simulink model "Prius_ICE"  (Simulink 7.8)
settings: Solver=ode23tb  StartTime=0.0  StopTime=1180  RelTol=1e-3
InitFcn:
  | init_Prius_GT
StopFcn:
  | Vyhodnoceni
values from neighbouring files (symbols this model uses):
  om_diff_ic = 0    [init_Prius_GT.m]
  omric = 0    [init_Prius_GT.m]
  rpm_FMEP = [1,500,1000,1500,2000,2500,3000,3500,4000,4500,5000]    [init_Prius_GT.m]
  t_sample = 0.1    [init_Prius_GT.m]
  torque_FMEP = [0,0,0.58,0.66,0.75,0.84,0.93,1.1,1.3,1.4,1.5].*(Vdis/(4*pi))*100000    [init_Prius_GT.m]
  vf0 = 0    [init_Prius_GT.m]
undefined symbols (not defined in the file or in its folder): Clutch, Control, Differential, Driveshaft, Engine, Environment, Gearbox, Powertrain, table_FMEP, Vehicle
libraries: simulink x30, simulink_extras x6, simulink_need_slupdate x1
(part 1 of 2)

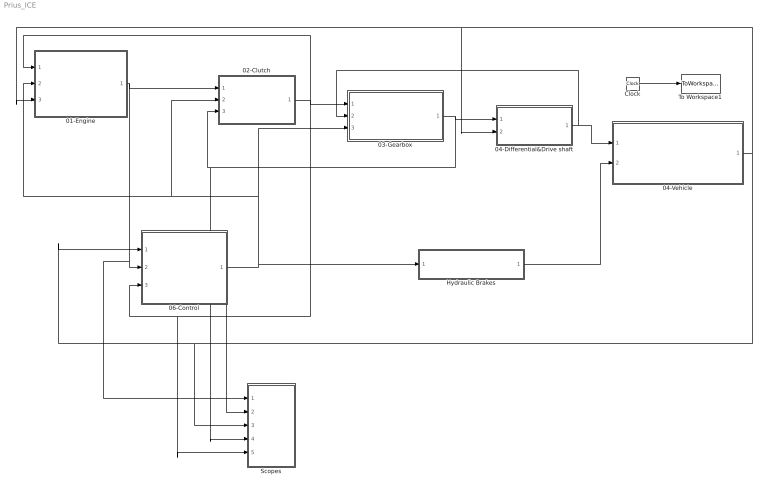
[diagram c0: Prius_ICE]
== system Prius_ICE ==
  01-Engine : Subsystem  AncestorBlock=Powertrain/01-Engine
  02-Clutch : Subsystem  AncestorBlock=Powertrain/02-Clutch
  03-Gearbox : Subsystem  AncestorBlock=Powertrain/03-Gearbox
  04-Differential&Drive shaft : Subsystem  AncestorBlock=Powertrain/04-Differential&Drive shaft
  04-Vehicle : Subsystem  AncestorBlock=Powertrain/05-Vehicle
  06-Control : Subsystem  AncestorBlock=Powertrain/06-Control
  Clock : Clock
  Hydraulic Brakes : Subsystem  AncestorBlock=Powertrain/Hydraulic Brakes  TreatAsAtomicUnit=on
  Scopes : Subsystem  AncestorBlock=Powertrain/Scopes
  To Workspace1 : ToWorkspace  VariableName=t  SampleTime=t_sample  SaveFormat=Array
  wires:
  01-Engine/1(BUS_Engine) -> 02-Clutch/1(BUS_Engine), 06-Control/2(BUS_Engine), Scopes/1(BUS_Engine)
  02-Clutch/1(BUS_Clutch) -> 03-Gearbox/1(BUS_Clutch), 01-Engine/1(BUS_Clutch), 06-Control/3(BUS_Clutch), Scopes/5(BUS_Clutch)
  03-Gearbox/1(BUS_Gearbox) -> 04-Differential&Drive shaft/1(BUS_Gearbox), 02-Clutch/3(BUS_Gearbox), Scopes/4(BUS_Gearbox)
  04-Differential&Drive shaft/1(BUS_Driveshaft) -> 03-Gearbox/2(BUS_Driveshaft), 04-Vehicle/1(BUS_Driveshaft_Front)
  06-Control/1(BUS_Control) -> Scopes/2(BUS_Control), 01-Engine/2(BUS_Control), 02-Clutch/2(BUS_Control), 03-Gearbox/3(BUS_Control), Hydraulic Brakes/1(BUS_Control)
  04-Vehicle/1(BUS_Vehicle) -> 06-Control/1(BUS_Vehicle), Scopes/3(BUS_Vehicle), 01-Engine/3(BUS_vehicle), 04-Differential&Drive shaft/2(BUS_Vehicle)
  Hydraulic Brakes/1(BUS_Brakes) -> 04-Vehicle/2(BUS_Brakes)
  Clock/1 -> To Workspace1/1

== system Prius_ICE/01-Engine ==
  note: Tec[Nm]
  BUS_Clutch : Inport
  BUS_Control : Inport  Port=2
  BUS_vehicle : Inport  Port=3
  1-D Lookup Table : Lookup_n-D  NumberOfTableDimensions=1  BreakpointsForDimension1=[1000,1625,2250,3000,3750,4500,5250,5625]  Table=[85,90,100,112,100,92,85,78]  RndMeth=Simplest
  Bus Creator : BusCreator  Inputs=5
  Bus Selector : BusSelector  OutputSignals=om_fric1
  Bus Selector1 : BusSelector  OutputSignals=Throttle_pedal[-],Status_Num
  Bus Selector2 : BusSelector  OutputSignals=s_veh
  Consumption/Emissions : Subsystem
  Display : Display
  Idling PID : Subsystem
  Mechanical1 : Subsystem
  Product2 : Product
  Saturation : Saturate  UpperLimit=inf  LowerLimit=0
  Scope : Scope  NumInputPorts=3
  rad2rpm : Gain  Gain=30/pi
  BUS_Engine : Outport
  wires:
  Idling PID/1(Te_dem) -> Mechanical1/1(Te_dem)
  1-D Lookup Table/1 -> Product2/1
  Product2/1 -> Idling PID/1(Te), Scope/3
  Bus Selector1/1 -> Scope/1, Product2/2  "<Throttle_pedal[-]>"
  Consumption/Emissions/2(Fuel_cons_m) -> Bus Creator/5  "Fuel_cons_m"
  Saturation/1 -> Consumption/Emissions/2(Pe)
  Consumption/Emissions/1(Fuel_cons) -> Bus Creator/4  "fuel_cons [l_100km]"
  Bus Selector2/1 -> Display/1, Consumption/Emissions/3(s)  "<s_veh>"
  BUS_vehicle/1 -> Bus Selector2/1
  BUS_Control/1 -> Bus Selector1/1
  Bus Selector/1 -> Mechanical1/2(om_fric)  "<om_fric1>"
  BUS_Clutch/1 -> Bus Selector/1
  Bus Creator/1 -> BUS_Engine/1
  Mechanical1/3(Tec) -> Bus Creator/3, Consumption/Emissions/4(Te)
  Mechanical1/2(Pe) -> Saturation/1, Bus Creator/2  "Pe[kW]"
  Mechanical1/1(om_e) -> rad2rpm/1
  rad2rpm/1 -> Scope/2, 1-D Lookup Table/1, Idling PID/2(n_eng[rpm]), Bus Creator/1, Consumption/Emissions/1(n_eng[rpm])  "n_eng[rpm]"

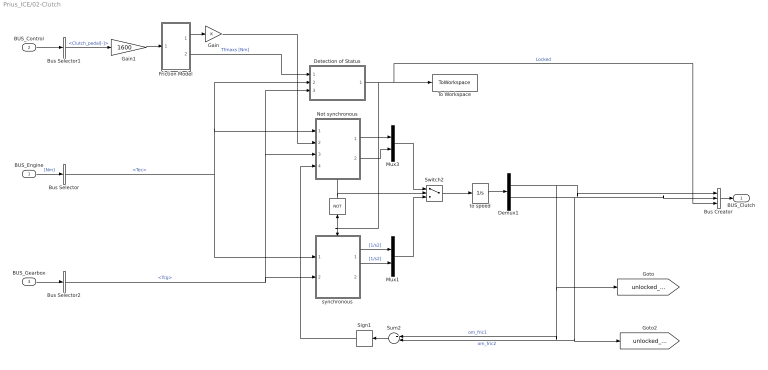
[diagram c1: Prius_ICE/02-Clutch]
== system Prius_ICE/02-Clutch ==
  BUS_Engine : Inport
  BUS_Control : Inport  Port=2
  BUS_Gearbox : Inport  Port=3
  " " : Logic  Operator=NOT  Inputs=1
  Bus Creator : BusCreator  Inputs=3
  Bus Selector : BusSelector  OutputSignals=Tec
  Bus Selector1 : BusSelector  OutputSignals=Clutch_pedal[-]
  Bus Selector2 : BusSelector  OutputSignals=Tcg
  Demux1 : Demux  Outputs=2
  Detection of Status : Subsystem
  Friction Model : Subsystem
  Gain : Gain
  Gain1 : Gain  Gain=1600
  Mux1 : Mux  Inputs=2
  Mux3 : Mux  Inputs=2
  Not synchronous : Subsystem  TreatAsAtomicUnit=on
  Sign1 : Signum
  Sum2 : Sum  Inputs=+-
  Switch2 : Switch  Threshold=0.5
  To Workspace : ToWorkspace  VariableName=ClutchLocked  SampleTime=t_sample  SaveFormat=Array
  synchronous : Subsystem  TreatAsAtomicUnit=on
  to speed : Integrator  InitialCondition=[0 0]
  BUS_Clutch : Outport
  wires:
  Gain/1 -> Not synchronous/2(Tfmaxk)
  Gain1/1 -> Friction Model/1(Fn)
  Bus Selector2/1 -> Detection of Status/3(T_cg), Not synchronous/3(T_cg), synchronous/2(T_cg)  "<Tcg>"
  BUS_Gearbox/1 -> Bus Selector2/1
  Bus Selector1/1 -> Gain1/1  "<Clutch_pedal[-]>"
  BUS_Control/1 -> Bus Selector1/1
  Bus Creator/1 -> BUS_Clutch/1
  Bus Selector/1 -> Detection of Status/2(T_ec), Not synchronous/1(T_ec), synchronous/1(T_ec)  "<Tec>"
  BUS_Engine/1 -> Bus Selector/1  "[Nm]"
  Friction Model/1(Tfmaxk) -> Gain/1
  Switch2/1 -> to speed/1
  to speed/1 -> Demux1/1
  Mux1/1 -> Switch2/3
  Mux3/1 -> Switch2/1
  Not synchronous/2(omp_c2) -> Mux3/2
  Sign1/1 -> Not synchronous/4(sign)
  Sum2/1 -> Sign1/1
  Not synchronous/1(omp_c1) -> Mux3/1
  Friction Model/2(Tfmaxs) -> Detection of Status/1(Tfmaxs)  "Tfmaxs [Nm]"
  Detection of Status/1(locked) -> Bus Creator/3, To Workspace/1, synchronous/Enable, " "/1  "Locked"
  " "/1 -> Not synchronous/Enable, Switch2/2
  Demux1/2 -> Bus Creator/2, [unlocked_wv], Sum2/2  "om_fric2"
  Demux1/1 -> Bus Creator/1, [unlocked_we], Sum2/1  "om_fric1"
  synchronous/2(omp_c2) -> Mux1/2  "[1/s2]"
  synchronous/1(omp_c1) -> Mux1/1  "[1/s2]"

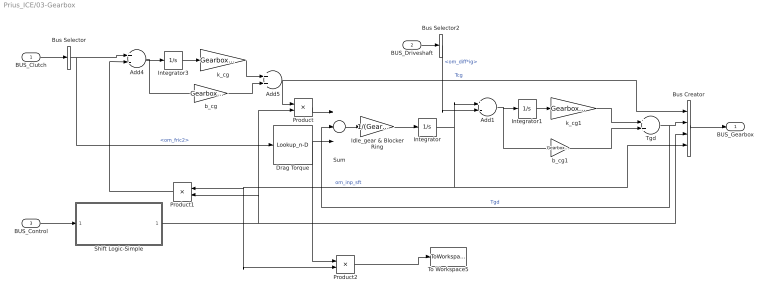
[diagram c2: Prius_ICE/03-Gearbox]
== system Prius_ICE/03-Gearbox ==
  BUS_Clutch : Inport
  BUS_Driveshaft : Inport  Port=2
  BUS_Control : Inport  Port=3
  Add1 : Sum  Inputs=+-
  Add4 : Sum  Inputs=+-
  Add5 : Sum
  Bus Creator : BusCreator
  Bus Selector : BusSelector  OutputSignals=om_fric2
  Bus Selector2 : BusSelector  OutputSignals=om_diff*ig
  Drag Torque : Lookup_n-D  NumberOfTableDimensions=1  BreakpointsForDimension1=[0 100 200 300 400]  Table=[0 1 2 3 3.5]  RndMeth=Simplest
  Idle_gear & Blocker Ring : Gain  Gain=1/(Gearbox.Inpsft.Inertia+Gearbox.Outpsft.Inertia)
  Integrator : Integrator
  Integrator1 : Integrator
  Integrator3 : Integrator
  Product : Product
  Product1 : Product
  Product2 : Product
  Shift Logic-Simple : Subsystem
  Sum : Sum  Inputs=+--
  Tgd : Sum
  To Workspace5 : ToWorkspace  VariableName=P_Gearbox  SampleTime=t_sample  SaveFormat=Array
  b_cg : Gain  Gain=Gearbox.Inpsft.b
  b_cg1 : Gain  Gain=Gearbox.Outpsft.b
  k_cg : Gain  Gain=Gearbox.Inpsft.c
  k_cg1 : Gain  Gain=Gearbox.Outpsft.c
  BUS_Gearbox : Outport
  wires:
  Drag Torque/1 -> Sum/3, Product2/1
  Bus Selector2/1 -> Add1/2  "<om_diff*ig>"
  BUS_Driveshaft/1 -> Bus Selector2/1
  Tgd/1 -> Bus Creator/2, Sum/2  "Tgd"
  Add1/1 -> b_cg1/1, Integrator1/1
  Integrator1/1 -> k_cg1/1
  k_cg1/1 -> Tgd/1
  b_cg1/1 -> Tgd/2
  Shift Logic-Simple/1(Gear_ratio) -> Bus Creator/3, Product1/2, Product/2
  Bus Creator/1 -> BUS_Gearbox/1
  BUS_Control/1 -> Shift Logic-Simple/1(BUS_Control)
  Bus Selector/1 -> Drag Torque/1, Add4/1  "<om_fric2>"
  BUS_Clutch/1 -> Bus Selector/1
  Product1/1 -> Add4/2
  Product/1 -> Sum/1
  b_cg/1 -> Add5/2
  k_cg/1 -> Add5/1
  Integrator3/1 -> k_cg/1
  Add4/1 -> Integrator3/1, b_cg/1
  Integrator/1 -> Add1/1, Bus Creator/4, Product1/1, Product2/2  "om_inp_sft"
  Idle_gear & Blocker Ring/1 -> Integrator/1
  Sum/1 -> Idle_gear & Blocker Ring/1
  Add5/1 -> Bus Creator/1, Product/1  "Tcg"
  Product2/1 -> To Workspace5/1

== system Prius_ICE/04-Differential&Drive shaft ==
  BUS_Gearbox : Inport
  BUS_Vehicle : Inport  Port=2
  Bus Creator : BusCreator  Inputs=2
  Bus Selector2 : BusSelector  OutputSignals=Tgd
  Differential : Subsystem
  Driveshafts : Subsystem
  BUS_Driveshaft : Outport
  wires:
  Driveshafts/1(T_drvsft) -> Differential/2(T_drv_sft), Bus Creator/1
  Differential/2(om_diff*ig) -> Bus Creator/2  "om_diff*ig"
  Bus Selector2/1 -> Differential/1(Tgd)  "<Tgd>"
  Differential/1(om_diff) -> Driveshafts/1(om_diff)
  BUS_Vehicle/1 -> Driveshafts/2(BUS_Vehicle)
  Bus Creator/1 -> BUS_Driveshaft/1
  BUS_Gearbox/1 -> Bus Selector2/1

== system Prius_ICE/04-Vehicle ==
  BUS_Driveshaft_Front : Inport
  BUS_Brakes : Inport  Port=2
  "          1" : Product  Inputs=**
  "          2" : Product  Inputs=**
  Add : Sum
  Bus Creator : BusCreator  Inputs=5
  Bus Selector1 : BusSelector  OutputSignals=T_drvsft
  Bus Selector3 : BusSelector  OutputSignals=Brakes_Front,Brakes_Rear
  Dynamics : Subsystem
  Subtract2 : Sum
  Tire front : Subsystem
  Tire rear : Subsystem
  To Workspace2 : ToWorkspace  VariableName=P_brakes  SampleTime=t_sample  SaveFormat=Array
  Weight distribution : Subsystem
  BUS_Vehicle : Outport
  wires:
  "          2"/1 -> Subtract2/2
  Subtract2/1 -> To Workspace2/1
  "          1"/1 -> Subtract2/1
  Bus Selector3/2 -> Tire rear/2(T_drsft), "          2"/2  "<Brakes_Rear>"
  Bus Selector3/1 -> "          1"/2, Add/2  "<Brakes_Front>"
  BUS_Brakes/1 -> Bus Selector3/1
  Bus Selector1/1 -> Add/1  "<T_drvsft>"
  Add/1 -> Tire front/2(T_drsft)
  Dynamics/2(s_veh) -> Bus Creator/2  "s_veh"
  Tire front/1(F_tire) -> Dynamics/1(F_tire_front)
  Tire rear/1(F_tire) -> Dynamics/2(F_tire_rear)
  BUS_Driveshaft_Front/1 -> Bus Selector1/1
  Bus Creator/1 -> BUS_Vehicle/1
  Weight distribution/1(Fn_Wheel_F) -> Dynamics/3(Fn_Wheel_F)
  Weight distribution/2(Fn_Wheel_R) -> Dynamics/4(Fn_Wheel_R)
  Dynamics/1(v_veh) -> Bus Creator/1  "v_veh"
  Dynamics/3(v_f[m/s]) -> Tire front/1(v_f), Tire rear/1(v_f)
  Dynamics/4(Acc) -> Bus Creator/5, Weight distribution/1(acc)  "a_veh"
  Tire front/2(om_wheel) -> "          1"/1, Bus Creator/3  "om_wheel_f"
  Tire rear/2(om_wheel) -> "          2"/1, Bus Creator/4  "om_wheel_r"

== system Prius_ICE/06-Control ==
  BUS_Vehicle : Inport
  BUS_Engine : Inport  Port=2
  BUS_Clutch : Inport  Port=3
  Bus Creator : BusCreator  Inputs=6
  Bus Selector : BusSelector  OutputSignals=n_eng[rpm]
  Bus Selector1 : BusSelector  OutputSignals=Locked,om_fric1
  Bus Selector2 : BusSelector  OutputSignals=v_veh
  Cockpit : Subsystem
  Cycle : Subsystem
  Driver : Subsystem
  Memory : Memory
  StateLogic : Subsystem  TreatAsAtomicUnit=on
  rad2rpm : Gain  Gain=30/pi
  BUS_Control : Outport
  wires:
  BUS_Engine/1 -> Bus Selector/1
  BUS_Clutch/1 -> Bus Selector1/1
  Bus Selector1/1 -> Memory/1  "<Locked>"
  Cockpit/2(Clutch1) -> Bus Creator/2  "Clutch_pedal[-]"
  StateLogic/1(Status_Num) -> Cockpit/1(Status_Num), Bus Creator/6, Driver/3(Status_Num)  "Status_Num"
  Cockpit/1(Throttle1) -> Bus Creator/1  "Throttle_pedal[-]"
  Cockpit/3(Brake1) -> Bus Creator/3  "Brake_pedal[-]"
  Driver/1(Throttle [Nm]) -> Cockpit/2(Throttle_in)
  Driver/2(Brake [Nm]) -> Cockpit/3(Brake)
  Cycle/2(v_dem [-]) -> Bus Creator/5, Driver/2(v_dem [km/h]), StateLogic/4(v_dem)  "v_dem[kmh]"
  Cycle/1(Gear_dem [-]) -> StateLogic/1(Gear), Bus Creator/4  "Gear[-]"
  Bus Creator/1 -> BUS_Control/1
  BUS_Vehicle/1 -> Bus Selector2/1
  Bus Selector2/1 -> StateLogic/2(v_veh), Driver/1(v_veh [km/h]), Cycle/1(v_veh [km/h])  "<v_veh>"
  Bus Selector1/2 -> rad2rpm/1  "<om_fric1>"
  Bus Selector/1 -> Driver/4(n_eng[rpm])  "<n_eng[rpm]>"
  Memory/1 -> StateLogic/3(Clutch_Locked)

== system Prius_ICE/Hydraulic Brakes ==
  BUS_Control : Inport
  Bus Creator : BusCreator  Inputs=2
  Bus Selector : BusSelector  OutputSignals=Brake_pedal[-]
  Gain1 : Gain  Gain=0.6
  Gain2 : Gain  Gain=0.4
  Pos2Nm : Gain  Gain=800
  BUS_Brakes : Outport
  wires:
  Pos2Nm/1 -> Gain2/1, Gain1/1
  Bus Creator/1 -> BUS_Brakes/1
  Gain2/1 -> Bus Creator/2  "Brakes_Rear"
  Gain1/1 -> Bus Creator/1  "Brakes_Front"
  BUS_Control/1 -> Bus Selector/1
  Bus Selector/1 -> Pos2Nm/1  "<Brake_pedal[-]>"

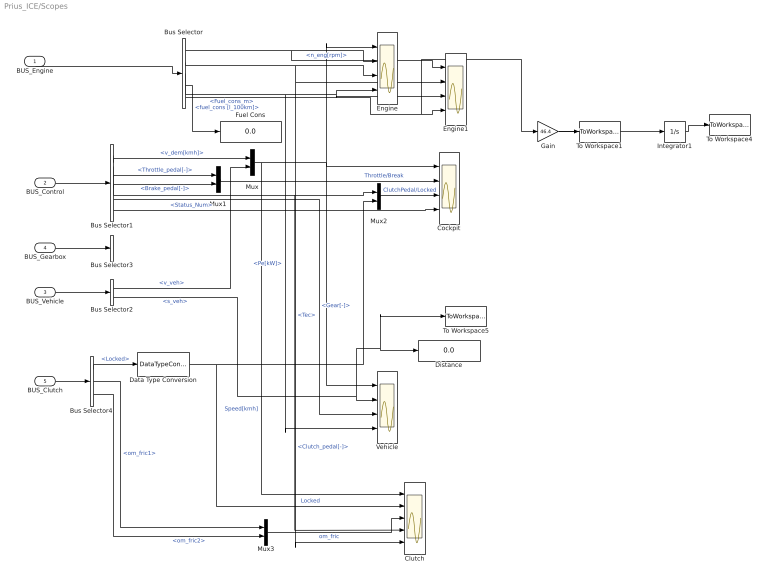
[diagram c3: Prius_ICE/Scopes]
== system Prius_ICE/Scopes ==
  BUS_Engine : Inport
  BUS_Control : Inport  Port=2
  BUS_Vehicle : Inport  Port=3
  BUS_Gearbox : Inport  Port=4
  BUS_Clutch : Inport  Port=5
  Bus Selector : BusSelector  OutputSignals=n_eng[rpm],Tec,Pe[kW],fuel_cons [l_100km],Fuel_cons_m
  Bus Selector1 : BusSelector  OutputSignals=v_dem[kmh],Throttle_pedal[-],Brake_pedal[-],Clutch_pedal[-],Gear[-],Status_Num
  Bus Selector2 : BusSelector  OutputSignals=v_veh,s_veh
  Bus Selector3 : BusSelector  OutputSignals=Gear_ratio [-]
  Bus Selector4 : BusSelector  OutputSignals=Locked,om_fric1,om_fric2
  Clutch : Scope  NumInputPorts=5
  Cockpit : Scope  NumInputPorts=4
  Data Type Conversion : DataTypeConversion
  Distance : Display
  Engine : Scope  NumInputPorts=4
  Engine1 : Scope  NumInputPorts=4
  Fuel Cons : Display
  Gain : Gain  Gain=46.4
  Integrator1 : Integrator
  Mux{,1..3} (4 alike) : Mux  Inputs=2
  To Workspace1 : ToWorkspace  VariableName=Pfuel  SampleTime=t_sample  SaveFormat=Array
  To Workspace4 : ToWorkspace  VariableName=Efuel  SampleTime=t_sample  SaveFormat=Array
  To Workspace5 : ToWorkspace  VariableName=s  SampleTime=t_sample  SaveFormat=Array
  Vehicle : Scope  NumInputPorts=4
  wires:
  BUS_Engine/1 -> Bus Selector/1
  BUS_Control/1 -> Bus Selector1/1
  BUS_Vehicle/1 -> Bus Selector2/1
  Bus Selector1/1 -> Mux/1  "<v_dem[kmh]>"
  Bus Selector2/1 -> Mux/2  "<v_veh>"
  Mux/1 -> Vehicle/1, Engine/1, Cockpit/1, Clutch/1  "Speed[kmh]"
  Bus Selector/1 -> Engine/2, Engine1/1  "<n_eng[rpm]>"
  Bus Selector/2 -> Engine/3, Engine1/2, Clutch/5  "<Tec>"
  Bus Selector/3 -> Vehicle/4, Engine/4, Engine1/3  "<Pe[kW]>"
  Bus Selector1/2 -> Mux1/1  "<Throttle_pedal[-]>"
  Bus Selector1/3 -> Mux1/2  "<Brake_pedal[-]>"
  Mux1/1 -> Cockpit/2  "Throttle/Break"
  Bus Selector2/2 -> Vehicle/2, Distance/1, To Workspace5/1  "<s_veh>"
  BUS_Gearbox/1 -> Bus Selector3/1
  Bus Selector1/5 -> Vehicle/3  "<Gear[-]>"
  BUS_Clutch/1 -> Bus Selector4/1
  Bus Selector1/4 -> Mux2/1, Clutch/4  "<Clutch_pedal[-]>"
  Bus Selector4/1 -> Data Type Conversion/1  "<Locked>"
  Mux2/1 -> Cockpit/3  "ClutchPedal/Locked"
  Data Type Conversion/1 -> Mux2/2, Clutch/2  "Locked"
  Mux3/1 -> Clutch/3  "om_fric"
  Bus Selector4/2 -> Mux3/1  "<om_fric1>"
  Bus Selector4/3 -> Mux3/2  "<om_fric2>"
  Bus Selector/4 -> Fuel Cons/1  "<fuel_cons [l_100km]>"
  Bus Selector/5 -> Engine1/4, Gain/1  "<Fuel_cons_m>"
  Bus Selector1/6 -> Cockpit/4  "<Status_Num>"
  Gain/1 -> To Workspace1/1, Integrator1/1
  Integrator1/1 -> To Workspace4/1

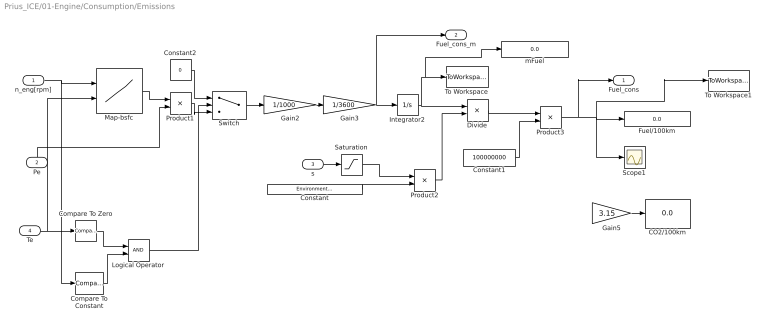
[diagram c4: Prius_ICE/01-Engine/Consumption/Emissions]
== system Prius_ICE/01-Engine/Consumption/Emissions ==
  n_eng[rpm] : Inport
  Pe : Inport  Port=2
  s : Inport  Port=3
  Te : Inport  Port=4
  CO2/100km : Display
  Compare To Constant : simulink/Logic and Bit Operations/Compare To Constant  relop=>=  const=2000  OutDataTypeStr=uint8
  Compare To Zero : simulink/Logic and Bit Operations/Compare To Zero  relop=<=  OutDataTypeStr=uint8
  Constant : Constant  Value=Environment.Fuel.ro
  Constant1 : Constant  Value=100000000
  Constant2 : Constant  Value=0
  Divide : Product  Inputs=*/
  Fuel/100km : Display
  Gain2 : Gain  Gain=1/1000
  Gain3 : Gain  Gain=1/3600
  Gain5 : Gain  Gain=3.15
  Integrator2 : Integrator
  Logical Operator : Logic  AllPortsSameDT=off  OutDataTypeStr=boolean
  Map-bsfc : Lookup2D  RowIndex=RPM  ColumnIndex=performance  Table=bsfc'  LookUpMeth=Interpolation-Use End Values
  Product1 : Product
  Product2 : Product
  Product3 : Product
  Saturation : Saturate  UpperLimit=inf  LowerLimit=10
  Scope1 : Scope
  Switch : Switch  Threshold=1
  To Workspace : ToWorkspace  VariableName=m_fuel  SampleTime=t_sample  SaveFormat=Array
  To Workspace1 : ToWorkspace  VariableName=fuel_cons_avg  SampleTime=t_sample  SaveFormat=Array
  mFuel : Display
  Fuel_cons : Outport
  Fuel_cons_m : Outport  Port=2
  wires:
  Constant2/1 -> Switch/1
  Switch/1 -> Gain2/1
  Product1/1 -> Switch/3
  Logical Operator/1 -> Switch/2
  Compare To Constant/1 -> Logical Operator/2
  Compare To Zero/1 -> Logical Operator/1
  Te/1 -> Compare To Zero/1, Map-bsfc/2
  Saturation/1 -> Product2/1
  Pe/1 -> Product1/2
  n_eng[rpm]/1 -> Compare To Constant/1, Map-bsfc/1
  Gain5/1 -> CO2/100km/1
  Product3/1 -> To Workspace1/1, Scope1/1, Fuel/100km/1, Fuel_cons/1
  Constant1/1 -> Product3/2
  Divide/1 -> Product3/1
  Product2/1 -> Divide/2
  Constant/1 -> Product2/2
  s/1 -> Saturation/1
  Integrator2/1 -> Divide/1, mFuel/1, To Workspace/1
  Gain3/1 -> Fuel_cons_m/1, Integrator2/1
  Gain2/1 -> Gain3/1
  Map-bsfc/1 -> Product1/1

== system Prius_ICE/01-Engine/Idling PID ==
  Te : Inport
  n_eng[rpm] : Inport  Port=2
  Add : Sum
  Add3 : Sum  Inputs=+-
  Compare To Zero : simulink/Logic and Bit Operations/Compare To Zero  relop=<=  OutDataTypeStr=uint8
  Constant2 : Constant  Value=0
  Data Type Conversion : DataTypeConversion
  Ground : Ground
  Idle rpm : Constant  Value=Engine.Idle.rpm
  PID Controller : simulink/Continuous/PID Controller  Controller=PID  TimeDomain=Continuous-time  SampleTime=1  IntegratorMethod=Forward Euler  FilterMethod=Forward Euler  Form=Parallel  P=10  I=0.001  D=0  N=100  InitialConditionSource=internal  InitialConditionForIntegrator=0  InitialConditionForFilter=0  ExternalReset=rising  LimitOutput=on  UpperSaturationLimit=200  LowerSaturationLimit=-inf  LinearizeAsGain=off  AntiWindupMode=none  Kb=1  TrackingMode=off  Kt=1  PParamMin=[]  PParamMax=[]  IParamMin=[]  IParamMax=[]  DParamMin=[]  DParamMax=[]  NParamMin=[]  NParamMax=[]  KbParamMin=[]  KbParamMax=[]  KtParamMin=[]  KtParamMax=[]  POutMin=[]  POutMax=[]  IOutMin=[]  IOutMax=[]  DOutMin=[]  DOutMax=[]  NOutMin=[]  NOutMax=[]  KbOutMin=[]  KbOutMax=[]  KtOutMin=[]  KtOutMax=[]  IntegratorOutMin=[]  IntegratorOutMax=[]  FilterOutMin=[]  FilterOutMax=[]  SumOutMin=[]  SumOutMax=[]  SumI1OutMin=[]  SumI1OutMax=[]  SumI2OutMin=[]  SumI2OutMax=[]  SumI3OutMin=[]  SumI3OutMax=[]  SumDOutMin=[]  SumDOutMax=[]  SaturationOutMin=[]  SaturationOutMax=[]  IntegratorContinuousStateAttributes=''  IntegratorStateMustResolveToSignalObject=off  IntegratorRTWStateStorageClass=Auto  FilterContinuousStateAttributes=''  FilterStateMustResolveToSignalObject=off  FilterRTWStateStorageClass=Auto
  Saturation1 : Saturate  UpperLimit=10  LowerLimit=0
  Scope : Scope  NumInputPorts=3
  Switch : Switch  Threshold=1
  Terminator_1 : Terminator
  Te_dem : Outport
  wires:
  Data Type Conversion/1 -> PID Controller/2
  Ground/1 -> Terminator_1/1
  Add/1 -> Te_dem/1
  n_eng[rpm]/1 -> Scope/3, Add3/2
  Constant2/1 -> Switch/3
  Switch/1 -> Scope/2, Add/2
  Saturation1/1 -> Switch/1
  Compare To Zero/1 -> Data Type Conversion/1, Switch/2
  Add3/1 -> PID Controller/1
  Idle rpm/1 -> Add3/1
  PID Controller/1 -> Saturation1/1
  Te/1 -> Scope/1, Add/1, Compare To Zero/1

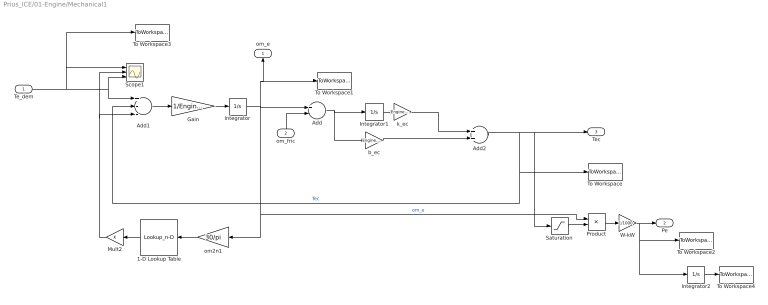
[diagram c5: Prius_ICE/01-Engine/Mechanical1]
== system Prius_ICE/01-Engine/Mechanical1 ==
  Te_dem : Inport
  om_fric : Inport  Port=2
  1-D Lookup Table : Lookup_n-D  NumberOfTableDimensions=1  BreakpointsForDimension1=rpm_FMEP  BreakpointsForDimension2=table_FMEP  Table=torque_FMEP  RndMeth=Simplest
  Add : Sum  Inputs=+-
  Add1 : Sum  Inputs=+--
  Add2 : Sum
  Gain : Gain  Gain=1/Engine.Inertia
  Integrator : Integrator
  Integrator1 : Integrator
  Integrator2 : Integrator
  Mult2 : Gain
  Product : Product
  Saturation : Saturate  UpperLimit=inf  LowerLimit=0
  Scope1 : Scope  NumInputPorts=3
  To Workspace : ToWorkspace  VariableName=Tengine_f  SampleTime=t_sample  SaveFormat=Array
  To Workspace1 : ToWorkspace  VariableName=om_e_f  SampleTime=t_sample  SaveFormat=Array
  To Workspace2 : ToWorkspace  VariableName=Pe  SampleTime=t_sample  SaveFormat=Array
  To Workspace3 : ToWorkspace  VariableName=Te_dem  SampleTime=t_sample  SaveFormat=Array
  To Workspace4 : ToWorkspace  VariableName=Eengine  SampleTime=t_sample  SaveFormat=Array
  W-kW : Gain  Gain=1/1000
  b_ec : Gain  Gain=Engine.Crankshaft.b
  k_ec : Gain  Gain=Engine.Crankshaft.c
  om2n1 : Gain  Gain=30/pi
  om_e : Outport
  Pe : Outport  Port=2
  Tec : Outport  Port=3
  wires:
  W-kW/1 -> Pe/1, Integrator2/1, To Workspace2/1
  Te_dem/1 -> Add1/1, Scope1/3, Scope1/1, To Workspace3/1
  b_ec/1 -> Add2/2
  k_ec/1 -> Add2/1
  Product/1 -> W-kW/1
  om_fric/1 -> Add/2
  Add2/1 -> Saturation/1, Tec/1, To Workspace/1, Add1/2  "Tec"
  Integrator1/1 -> k_ec/1
  Add/1 -> b_ec/1, Integrator1/1
  Integrator/1 -> To Workspace1/1, om_e/1, om2n1/1, Product/1, Add/1  "om_e"
  Gain/1 -> Integrator/1
  Add1/1 -> Gain/1
  Integrator2/1 -> To Workspace4/1
  1-D Lookup Table/1 -> Mult2/1
  om2n1/1 -> 1-D Lookup Table/1
  Mult2/1 -> Add1/3, Scope1/2
  Saturation/1 -> Product/2

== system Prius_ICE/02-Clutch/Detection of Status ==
  Tfmaxs : Inport
  T_ec : Inport  Port=2
  T_cg : Inport  Port=3
  Break Apart Detection : Subsystem
  Combinatorial  Logic : CombinatorialLogic  TruthTable=[0;1;0;0;1;1;1;0]
  Compare To Zero : simulink/Logic and Bit Operations/Compare To Zero  relop=<=  OutDataTypeStr=uint8
  Lockup Detection : Subsystem
  Memory : Memory
  Mux : Mux  Inputs=3
  Timer : Subsystem
  locked : Outport
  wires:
  Compare To Zero/1 -> Timer/1(Set)
  Timer/1(Count) -> Lockup Detection/4(Count)
  T_ec/1 -> Break Apart Detection/1(T_ec), Lockup Detection/1(T_ec)
  Lockup Detection/1(Lock Up) -> Mux/1  "lock"
  Mux/1 -> Combinatorial  Logic/1
  Memory/1 -> Mux/3
  Combinatorial  Logic/1 -> Compare To Zero/1, locked/1, Memory/1
  Break Apart Detection/1(Break Apart) -> Mux/2  "unlock"
  T_cg/1 -> Lockup Detection/2(T_cg), Break Apart Detection/2(T_cg)
  Tfmaxs/1 -> Lockup Detection/3(Tfmaxs), Break Apart Detection/3(Tfmaxs)

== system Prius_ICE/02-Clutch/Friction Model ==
  Fn : Inport
  Ratio of static to kinetic : Gain  Gain=Clutch.mus/Clutch.muk
  Torque Conversion : Gain  Gain=2/3*Clutch.Radius*Clutch.muk
  Tfmaxk : Outport  InitialOutput=0
  Tfmaxs : Outport  Port=2  InitialOutput=0
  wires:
  Ratio of static to kinetic/1 -> Tfmaxs/1
  Fn/1 -> Torque Conversion/1
  Torque Conversion/1 -> Ratio of static to kinetic/1, Tfmaxk/1

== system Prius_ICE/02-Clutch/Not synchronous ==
  T_ec : Inport
  Tfmaxk : Inport  Port=2
  T_cg : Inport  Port=3
  sign : Inport  Port=4
  Enable : EnablePort  StatesWhenEnabling=reset  PropagateVarSize=During execution
  Inertia : Gain  Gain=1/Clutch.Inp.Inertia
  Inertia1 : Gain  Gain=1/Clutch.Out.Inertia
  Mux : Mux  Inputs=2
  Product : Product
  Scope : Scope  NumInputPorts=2
  Scope1 : Scope
  Sum : Sum  Inputs=+|-
  Sum1 : Sum  Inputs=+|-
  omp_c1 : Outport
  omp_c2 : Outport  Port=2
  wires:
  Mux/1 -> Scope1/1
  T_ec/1 -> Sum/1  "T_ec"
  sign/1 -> Product/2
  Inertia1/1 -> omp_c2/1  "omp_c2[rad/s2]"
  T_cg/1 -> Sum1/2  "T_cg"
  Inertia/1 -> omp_c1/1  "omp_c1[rad/s2]"
  Tfmaxk/1 -> Product/1  "Tfmaxk"
  Product/1 -> Sum1/1, Sum/2  "sign(om_idle-om_blk)* T_cone"
  Sum/1 -> Mux/1, Scope/1, Inertia/1
  Sum1/1 -> Mux/2, Scope/2, Inertia1/1

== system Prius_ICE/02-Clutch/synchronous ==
  T_ec : Inport
  T_cg : Inport  Port=2
  Enable : EnablePort  StatesWhenEnabling=reset  PropagateVarSize=During execution
  Idle_gear & Blocker Ring : Gain  Gain=1/(Clutch.Inp.Inertia+Clutch.Out.Inertia)
  Scope1 : Scope
  Sum : Sum  Inputs=+|-
  omp_c1 : Outport
  omp_c2 : Outport  Port=2
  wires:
  T_ec/1 -> Sum/1
  T_cg/1 -> Sum/2
  Idle_gear & Blocker Ring/1 -> Scope1/1, omp_c2/1, omp_c1/1  "[rad/s2]"
  Sum/1 -> Idle_gear & Blocker Ring/1

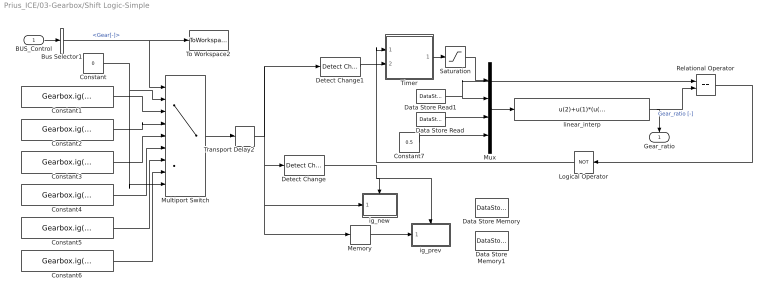
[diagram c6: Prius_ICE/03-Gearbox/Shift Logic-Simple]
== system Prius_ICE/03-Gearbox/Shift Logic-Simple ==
  BUS_Control : Inport
  Bus Selector1 : BusSelector  OutputSignals=Gear[-]
  Constant : Constant  Value=0
  Constant1 : Constant  Value=Gearbox.ig(1)
  Constant2 : Constant  Value=Gearbox.ig(2)
  Constant3 : Constant  Value=Gearbox.ig(3)
  Constant4 : Constant  Value=Gearbox.ig(4)
  Constant5 : Constant  Value=Gearbox.ig(5)
  Constant6 : Constant  Value=Gearbox.ig(6)
  Constant7 : Constant  Value=0.5
  Data Store Memory : DataStoreMemory  DataStoreName=ig_new
  Data Store Memory1 : DataStoreMemory  DataStoreName=ig_prev
  Data Store Read : DataStoreRead  DataStoreName=ig_new  SampleTime=0
  Data Store Read1 : DataStoreRead  DataStoreName=ig_prev  SampleTime=0
  Detect Change : simulink/Logic and Bit Operations/Detect Change  vinit=0  InputProcessing=Inherited  OutDataTypeStr=uint8
  Detect Change1 : simulink/Logic and Bit Operations/Detect Change  vinit=0  InputProcessing=Inherited  OutDataTypeStr=boolean
  Logical Operator : Logic  Operator=NOT  AllPortsSameDT=off  OutDataTypeStr=boolean
  Memory : Memory
  Multiport Switch : MultiPortSwitch  DataPortOrder=Zero-based contiguous  Inputs=7  DataPortForDefault=Additional data port  zeroidx=on
  Mux : Mux
  Relational Operator : RelationalOperator  Operator===  OutDataTypeStr=boolean
  Saturation : Saturate  LowerLimit=0
  Timer : Subsystem
  To Workspace2 : ToWorkspace  VariableName=Gear  SampleTime=t_sample  SaveFormat=Array
  Transport Delay2 : TransportDelay  DelayTime=0.3  BufferSize=10000
  ig_new : Subsystem  TreatAsAtomicUnit=on
  ig_prev : Subsystem  TreatAsAtomicUnit=on
  linear_interp : Fcn  Expr=u(2)+u(1)*(u(3)-u(2))/u(4)
  Gear_ratio : Outport
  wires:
  BUS_Control/1 -> Bus Selector1/1
  Transport Delay2/1 -> Detect Change1/1, Memory/1, ig_new/1(ig), Detect Change/1
  Saturation/1 -> Mux/1
  Logical Operator/1 -> Timer/1(Set)
  Detect Change1/1 -> Timer/2(Reset)
  Relational Operator/1 -> Logical Operator/1
  linear_interp/1 -> Gear_ratio/1, Relational Operator/2  "Gear_ratio [-]"
  Constant7/1 -> Mux/4
  Data Store Read/1 -> Mux/3
  Data Store Read1/1 -> Mux/2, Relational Operator/1
  Timer/1(Count) -> Saturation/1
  Memory/1 -> ig_prev/1(ig)
  Detect Change/1 -> ig_prev/Trigger, ig_new/Trigger
  Mux/1 -> linear_interp/1
  Constant/1 -> Multiport Switch/9, Multiport Switch/2
  Constant6/1 -> Multiport Switch/8
  Constant5/1 -> Multiport Switch/7
  Constant4/1 -> Multiport Switch/6
  Constant3/1 -> Multiport Switch/5
  Constant2/1 -> Multiport Switch/4
  Constant1/1 -> Multiport Switch/3
  Bus Selector1/1 -> Multiport Switch/1, To Workspace2/1  "<Gear[-]>"
  Multiport Switch/1 -> Transport Delay2/1

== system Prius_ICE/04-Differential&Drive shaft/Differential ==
  Tgd : Inport
  T_drv_sft : Inport  Port=2
  Gain : Gain  Gain=Differential.ig(1)
  Sum5 : Sum  Inputs=+-|
  inertia rear drive shaft : Gain  Gain=1/Differential.Inertia
  ratio target gear : Gain  Gain=Differential.ig(1)
  "to_angle " : Integrator  InitialCondition=om_diff_ic
  om_diff : Outport
  om_diff*ig : Outport  Port=2
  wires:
  Gain/1 -> om_diff*ig/1
  Tgd/1 -> ratio target gear/1
  ratio target gear/1 -> Sum5/1  "T_outp_sft_i"
  "to_angle "/1 -> Gain/1, om_diff/1  "om_diff [rad/s]"
  Sum5/1 -> inertia rear drive shaft/1
  inertia rear drive shaft/1 -> "to_angle "/1  "omp_diff"
  T_drv_sft/1 -> Sum5/2  "T_drv_sft"

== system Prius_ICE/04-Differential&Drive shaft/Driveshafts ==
  om_diff : Inport
  BUS_Vehicle : Inport  Port=2
  Add4 : Sum  Inputs=+-
  Add5 : Sum
  Bus Selector1 : BusSelector  OutputSignals=om_wheel_f
  Integrator3 : Integrator
  To Workspace1 : ToWorkspace  VariableName=T_drvsft  SampleTime=t_sample  SaveFormat=Array
  b_cg : Gain  Gain=Driveshaft.Left.b+Driveshaft.Right.b
  k_cg : Gain  Gain=Driveshaft.Left.c+Driveshaft.Right.c
  T_drvsft : Outport
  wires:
  BUS_Vehicle/1 -> Bus Selector1/1
  om_diff/1 -> Add4/1
  Add5/1 -> T_drvsft/1, To Workspace1/1  "T_drvsft"
  b_cg/1 -> Add5/2
  k_cg/1 -> Add5/1
  Integrator3/1 -> k_cg/1
  Add4/1 -> Integrator3/1, b_cg/1
  Bus Selector1/1 -> Add4/2  "<om_wheel_f>"

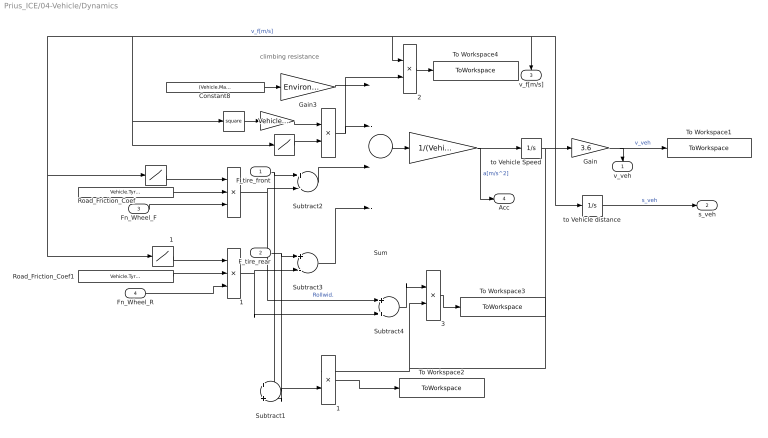
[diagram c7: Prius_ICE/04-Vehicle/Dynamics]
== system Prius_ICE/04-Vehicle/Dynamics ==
  note: climbing resistance
  F_tire_front : Inport
  F_tire_rear : Inport  Port=2
  Fn_Wheel_F : Inport  Port=3
  Fn_Wheel_R : Inport  Port=4
  "  " : Gain  Gain=1/(Vehicle.Mass+Vehicle.Load)
  "     " : Gain  Gain=Vehicle.cx*Vehicle.AreaF*Environment.Air.ro*0.5
  "      " : Math  Operator=square
  "        " : Product  Inputs=***
  "         " : Lookup  InputValues=[-1 -0.01 0 0.01 1]  Table=[-1 -1 0 1 1]
            {,1..3} (4 alike) : Product  Inputs=**
  "            " : Lookup  InputValues=[-1 -0.01 0 0.01 1]  Table=[-1 -1 0 1 1]
  "         1" : Lookup  InputValues=[-1 -0.01 0 0.01 1]  Table=[-1 -1 0 1 1]
  "        1" : Product  Inputs=***
  Constant8 : Constant  Value=(Vehicle.Mass+Vehicle.Load)
  Gain : Gain  Gain=3.6
  Gain3 : Gain  Gain=Environment.g*sin(Environment.Road.Incline)
  Road_Friction_Coef : Constant  Value=Vehicle.Tyre.Front.f
  Road_Friction_Coef1 : Constant  Value=Vehicle.Tyre.Rear.f
  Subtract1 : Sum
  Subtract2 : Sum  Inputs=+-
  Subtract3 : Sum  Inputs=+-
  Subtract4 : Sum
  Sum : Sum  Inputs=|-|-|+|+
  To Workspace1 : ToWorkspace  VariableName=v_vehicle  SampleTime=t_sample  SaveFormat=Array
  To Workspace2 : ToWorkspace  VariableName=P_vehicle  SampleTime=t_sample  SaveFormat=Array
  To Workspace3 : ToWorkspace  VariableName=P_roll  SampleTime=t_sample  SaveFormat=Array
  To Workspace4 : ToWorkspace  VariableName=P_air  SampleTime=t_sample  SaveFormat=Array
  to Vehicle Speed : Integrator  InitialCondition=vf0
  to Vehicle distance : Integrator  InitialCondition=vf0
  v_veh : Outport
  s_veh : Outport  Port=2
  v_f[m/s] : Outport  Port=3
  Acc : Outport  Port=4
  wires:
  "          3"/1 -> To Workspace3/1
  Subtract4/1 -> "          3"/1
  "          2"/1 -> To Workspace4/1
  Subtract1/1 -> "          1"/2
  "          1"/1 -> To Workspace2/1
  Sum/1 -> "  "/1
  "      "/1 -> "     "/1
  "         "/1 -> "        "/1
  Road_Friction_Coef/1 -> "        "/2
  "          "/1 -> "          2"/2, Sum/2
  "     "/1 -> "          "/1
  "            "/1 -> "          "/2
  "  "/1 -> to Vehicle Speed/1, Acc/1  "a[m/s^2]"
  to Vehicle Speed/1 -> "          3"/2, "          1"/1, Gain/1, to Vehicle distance/1, "          2"/1, "      "/1, "            "/1, "         "/1, "         1"/1, v_f[m/s]/1  "v_f[m/s]"
  Gain/1 -> To Workspace1/1, v_veh/1  "v_veh"
  Subtract2/1 -> Sum/3
  "        "/1 -> Subtract4/1, Subtract2/2  "Rollwid."
  "         1"/1 -> "        1"/1
  Road_Friction_Coef1/1 -> "        1"/2
  Subtract3/1 -> Sum/4
  "        1"/1 -> Subtract4/2, Subtract3/2
  Constant8/1 -> Gain3/1
  Gain3/1 -> Sum/1
  to Vehicle distance/1 -> s_veh/1  "s_veh"
  F_tire_front/1 -> Subtract1/1, Subtract2/1
  Fn_Wheel_F/1 -> "        "/3
  F_tire_rear/1 -> Subtract1/2, Subtract3/1
  Fn_Wheel_R/1 -> "        1"/3

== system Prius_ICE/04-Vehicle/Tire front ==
  v_f : Inport
  T_drsft : Inport  Port=2
  "            " : Gain  Gain=2
  "            1" : Gain  Gain=Vehicle.Tyre.Front.c
  "            2" : Gain  Gain=Vehicle.Tyre.Front.Rdyn
  "            3" : Gain  Gain=Vehicle.Tyre.Front.b
  Sum1 : Sum  Inputs=2
  Sum10 : Sum  Inputs=+-
  To Workspace1 : ToWorkspace  VariableName=om_wheel  SampleTime=t_sample  SaveFormat=Array
  Wheel : Subsystem
  "to Rot Speed     " : Integrator
  F_tire : Outport
  om_wheel : Outport  Port=2
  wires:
  T_drsft/1 -> Wheel/2(T_drsft)  "T_drv_sft"
  "            "/1 -> F_tire/1  "F_tire [N]"
  Sum1/1 -> "            "/1, Wheel/1(F_tire)  "[N]"
  Wheel/1(om_wheel) -> "            2"/1, om_wheel/1, To Workspace1/1  "om_wheel [1/s]"
  v_f/1 -> Sum10/2
  "to Rot Speed     "/1 -> "            1"/1
  "            2"/1 -> Sum10/1
  Sum10/1 -> "to Rot Speed     "/1, "            3"/1
  "            1"/1 -> Sum1/1  "[N]"
  "            3"/1 -> Sum1/2

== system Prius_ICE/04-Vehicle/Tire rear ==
  v_f : Inport
  T_drsft : Inport  Port=2
  "            " : Gain  Gain=2
  "            1" : Gain  Gain=Vehicle.Tyre.Front.c
  "            2" : Gain  Gain=Vehicle.Tyre.Front.Rdyn
  "            3" : Gain  Gain=Vehicle.Tyre.Front.b
  Sum1 : Sum  Inputs=2
  Sum10 : Sum  Inputs=+-
  To Workspace1 : ToWorkspace  VariableName=om_wheel2  SampleTime=t_sample  SaveFormat=Array
  Wheel : Subsystem
  "to Rot Speed     " : Integrator
  F_tire : Outport
  om_wheel : Outport  Port=2
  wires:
  "            3"/1 -> Sum1/2
  "            1"/1 -> Sum1/1  "[N]"
  Sum10/1 -> "            3"/1, "to Rot Speed     "/1
  "            2"/1 -> Sum10/1
  "to Rot Speed     "/1 -> "            1"/1
  v_f/1 -> Sum10/2
  Wheel/1(om_wheel) -> "            2"/1, To Workspace1/1, om_wheel/1  "om_wheel [1/s]"
  Sum1/1 -> Wheel/1(F_tire), "            "/1  "[N]"
  "            "/1 -> F_tire/1  "F_tire [N]"
  T_drsft/1 -> Wheel/2(T_drsft)  "T_drv_sft"

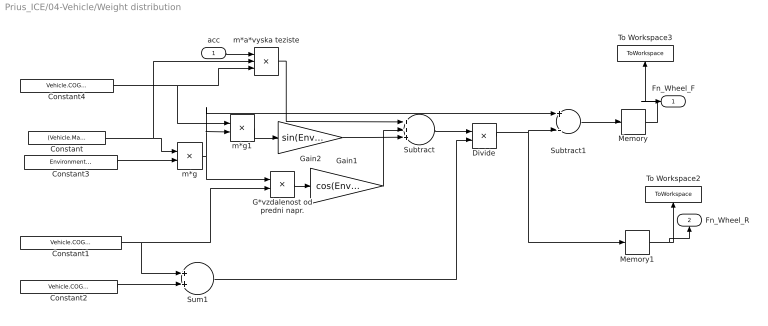
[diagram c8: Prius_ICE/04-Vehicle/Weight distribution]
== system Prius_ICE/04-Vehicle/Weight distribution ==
  acc : Inport
  Constant : Constant  Value=(Vehicle.Mass+Vehicle.Load)
  Constant1 : Constant  Value=Vehicle.COG.Front
  Constant2 : Constant  Value=Vehicle.COG.Rear
  Constant3 : Constant  Value=Environment.g
  Constant4 : Constant  Value=Vehicle.COG.Height
  Divide : Product  Inputs=*/
  G*vzdalenost od predni napr. : Product
  Gain1 : Gain  Gain=cos(Environment.Road.Incline)
  Gain2 : Gain  Gain=sin(Environment.Road.Incline)
  Memory : Memory  X0=Vehicle.Mass/2
  Memory1 : Memory  X0=Vehicle.Mass/2
  Subtract : Sum  Inputs=+++
  Subtract1 : Sum  Inputs=+-
  Sum1 : Sum
  To Workspace2 : ToWorkspace  VariableName=Fn_Wheel_R  SampleTime=t_sample  SaveFormat=Array
  To Workspace3 : ToWorkspace  VariableName=Fn_Wheel_F  SampleTime=t_sample  SaveFormat=Array
  m*a*vyska teziste : Product  Inputs=3
  m*g : Product
  m*g1 : Product
  Fn_Wheel_F : Outport
  Fn_Wheel_R : Outport  Port=2
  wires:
  Subtract1/1 -> Memory/1
  Divide/1 -> Subtract1/2, Memory1/1
  Subtract/1 -> Divide/1
  m*g/1 -> G*vzdalenost od predni napr./1, Subtract1/1, m*g1/2
  G*vzdalenost od predni napr./1 -> Gain1/1
  m*a*vyska teziste/1 -> Subtract/1
  Constant4/1 -> m*a*vyska teziste/3, m*g1/1
  Sum1/1 -> Divide/2
  Constant2/1 -> Sum1/2
  Constant1/1 -> Sum1/1, G*vzdalenost od predni napr./2
  Constant3/1 -> m*g/2
  Constant/1 -> m*g/1, m*a*vyska teziste/2
  Memory/1 -> To Workspace3/1, Fn_Wheel_F/1
  Memory1/1 -> To Workspace2/1, Fn_Wheel_R/1
  Gain1/1 -> Subtract/2
  m*g1/1 -> Gain2/1
  Gain2/1 -> Subtract/3
  acc/1 -> m*a*vyska teziste/1

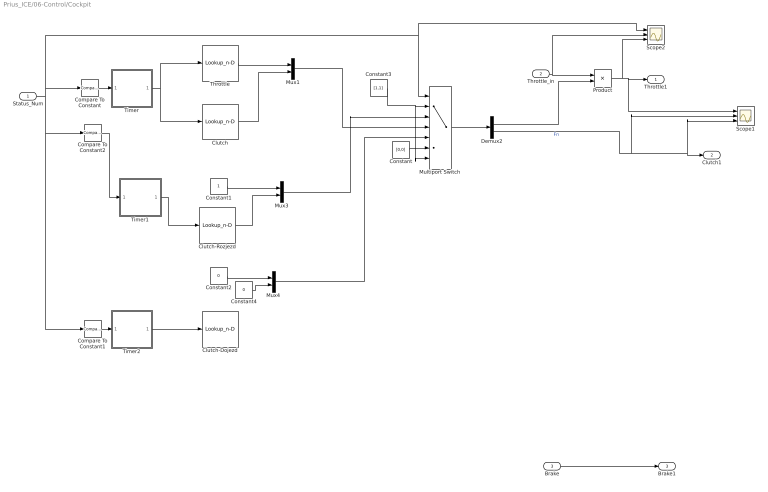
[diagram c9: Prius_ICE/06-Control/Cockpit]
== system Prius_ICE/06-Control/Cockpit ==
  Status_Num : Inport
  Throttle_in : Inport  Port=2
  Brake : Inport  Port=3
  Clutch : Lookup_n-D  NumberOfTableDimensions=1  BreakpointsForDimension1=[0 0.2 0.3 0.9 1.0 1.2]  Table=[1 1 0 0 1 1]  RndMeth=Simplest
  Clutch-Dojezd : Lookup_n-D  NumberOfTableDimensions=1  BreakpointsForDimension1=[0 0.05 0.3 1.9 2]  Table=[1 0 0 0 0]  ExtrapMethod=Clip  UseLastTableValue=on  RndMeth=Simplest
  Clutch-Rozjezd : Lookup_n-D  NumberOfTableDimensions=1  BreakpointsForDimension1=[0,0.5,0.6,1.1,1.4,1.5]  Table=[0,0,0.05,0.2,0.5,1]  ExtrapMethod=Clip  UseLastTableValue=on  RndMeth=Simplest
  Compare To Constant : simulink/Logic and Bit Operations/Compare To Constant  relop===  const=2  OutDataTypeStr=uint8
  Compare To Constant1 : simulink/Logic and Bit Operations/Compare To Constant  relop===  const=3  OutDataTypeStr=uint8
  Compare To Constant2 : simulink/Logic and Bit Operations/Compare To Constant  relop===  const=1  OutDataTypeStr=uint8
  Constant : Constant  Value=[0,0]
  Constant1 : Constant
  Constant2 : Constant  Value=0
  Constant3 : Constant  Value=[1,1]
  Constant4 : Constant  Value=0
  Demux2 : Demux  Outputs=2
  Multiport Switch : MultiPortSwitch  DataPortOrder=Zero-based contiguous  Inputs=5  DataPortForDefault=Additional data port  zeroidx=on
  Mux1 : Mux  Inputs=2
  Mux3 : Mux  Inputs=2
  Mux4 : Mux  Inputs=2
  Product : Product
  Scope1 : Scope  NumInputPorts=3
  Scope2 : Scope  NumInputPorts=3
  Throttle : Lookup_n-D  NumberOfTableDimensions=1  BreakpointsForDimension1=[0 0.1 0.2 1 1.1 1.2]  Table=[1 1 0 0 1 1]  RndMeth=Simplest
  Timer : Subsystem
  Timer1 : Subsystem
  Timer2 : Subsystem
  Throttle1 : Outport
  Clutch1 : Outport  Port=2
  Brake1 : Outport  Port=3
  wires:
  Timer/1(Count) -> Throttle/1, Clutch/1
  Throttle/1 -> Mux1/1
  Clutch/1 -> Mux1/2
  Demux2/2 -> Scope1/2, Clutch1/1, Scope1/3  "Fn"
  Constant1/1 -> Mux3/1
  Timer2/1(Count) -> Clutch-Dojezd/1
  Constant2/1 -> Mux4/1
  Multiport Switch/1 -> Demux2/1
  Status_Num/1 -> Compare To Constant2/1, Compare To Constant1/1, Compare To Constant/1, Multiport Switch/1, Scope2/1
  Constant3/1 -> Multiport Switch/2, Multiport Switch/7
  Mux3/1 -> Multiport Switch/3
  Mux1/1 -> Multiport Switch/4
  Mux4/1 -> Multiport Switch/5
  Constant/1 -> Multiport Switch/6
  Compare To Constant/1 -> Timer/1(Set)
  Compare To Constant1/1 -> Timer2/1(Set)
  Product/1 -> Throttle1/1, Scope1/1, Scope2/3
  Demux2/1 -> Product/2
  Throttle_in/1 -> Product/1, Scope2/2
  Brake/1 -> Brake1/1
  Clutch-Rozjezd/1 -> Mux3/2
  Compare To Constant2/1 -> Timer1/1(Set)
  Timer1/1(Count) -> Clutch-Rozjezd/1
  Constant4/1 -> Mux4/2

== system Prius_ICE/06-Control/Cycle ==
  v_veh [km/h] : Inport
  1-D Lookup Table : Lookup_n-D  NumberOfTableDimensions=1  BreakpointsForDimension1=[-5 0 0.1 30 30.5 45 45.5 65 65.5 85 85.5 200]  Table=[0 0 1 1 2 2 3 3 4 4 5 5]  InterpMethod=Flat  RndMeth=Simplest
  Cockpit : Scope  NumInputPorts=4
  Demux : Demux  Outputs=2
  Demux1 : Demux  Outputs=2
  From File : FromFile  FileName=NEDC.mat  ExtrapolationBeforeFirstDataPoint=Hold first value  ExtrapolationAfterLastDataPoint=Hold last value  SampleTime=0.1
  From File1 : FromFile  FileName=NEDC.mat  ExtrapolationBeforeFirstDataPoint=Hold first value  InterpolationWithinTimeRange=Zero order hold  ExtrapolationAfterLastDataPoint=Hold last value  SampleTime=0.1
  From File2 : FromFile  FileName=artemis_URM150.mat  ExtrapolationBeforeFirstDataPoint=Hold first value  ExtrapolationAfterLastDataPoint=Hold last value  SampleTime=0.1
  Terminator : Terminator
  Terminator1 : Terminator
  To Workspace : ToWorkspace  VariableName=v_dem  SampleTime=t_sample  SaveFormat=Array
  To Workspace2 : ToWorkspace  VariableName=Gear_dem  SampleTime=t_sample  SaveFormat=Array
  Gear_dem [-] : Outport
  v_dem [-] : Outport  Port=2
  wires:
  From File/1 -> Demux/1
  Demux/2 -> Terminator/1
  From File1/1 -> Demux1/1
  Demux1/1 -> Terminator1/1
  From File2/1 -> 1-D Lookup Table/1
  Demux1/2 -> To Workspace2/1, Gear_dem [-]/1
  Demux/1 -> To Workspace/1, v_dem [-]/1

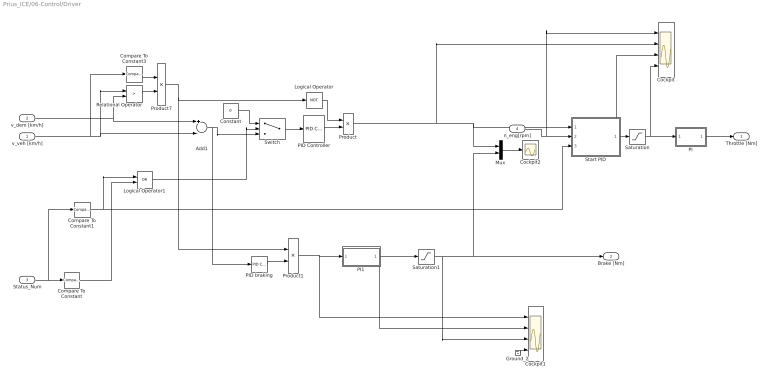
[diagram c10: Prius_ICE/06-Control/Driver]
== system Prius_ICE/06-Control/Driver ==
  v_veh [km/h] : Inport
  v_dem [km/h] : Inport  Port=2
  Status_Num : Inport  Port=3
  n_eng[rpm] : Inport  Port=4
  Add1 : Sum  Inputs=+-
  Cockpit : Scope  NumInputPorts=4
  Cockpit1 : Scope  NumInputPorts=4
  Cockpit2 : Scope
  Compare To Constant : simulink/Logic and Bit Operations/Compare To Constant  relop===  const=2  OutDataTypeStr=uint8
  Compare To Constant1 : simulink/Logic and Bit Operations/Compare To Constant  relop===  const=1  OutDataTypeStr=boolean
  Compare To Constant3 : simulink/Logic and Bit Operations/Compare To Constant  relop=>  const=1  OutDataTypeStr=uint8  ZeroCross=off
  Constant : Constant  Value=0
  Ground_2 : Ground
  Logical Operator : Logic  Operator=NOT  AllPortsSameDT=off  OutDataTypeStr=boolean
  Logical Operator1 : Logic  Operator=OR  AllPortsSameDT=off  OutDataTypeStr=boolean
  Mux : Mux  Inputs=2
  PI : Subsystem
  PI1 : Subsystem
  PID Controller : simulink/Continuous/PID Controller  Controller=PID  TimeDomain=Continuous-time  SampleTime=1  IntegratorMethod=Forward Euler  FilterMethod=Forward Euler  Form=Parallel  P=0.2  I=0.001  D=0  N=100  InitialConditionSource=internal  InitialConditionForIntegrator=0  InitialConditionForFilter=0  ExternalReset=none  LimitOutput=on  UpperSaturationLimit=1  LowerSaturationLimit=0  LinearizeAsGain=off  AntiWindupMode=none  Kb=1  TrackingMode=off  Kt=1  PParamMin=[]  PParamMax=[]  IParamMin=[]  IParamMax=[]  DParamMin=[]  DParamMax=[]  NParamMin=[]  NParamMax=[]  KbParamMin=[]  KbParamMax=[]  KtParamMin=[]  KtParamMax=[]  POutMin=[]  POutMax=[]  IOutMin=[]  IOutMax=[]  DOutMin=[]  DOutMax=[]  NOutMin=[]  NOutMax=[]  KbOutMin=[]  KbOutMax=[]  KtOutMin=[]  KtOutMax=[]  IntegratorOutMin=[]  IntegratorOutMax=[]  FilterOutMin=[]  FilterOutMax=[]  SumOutMin=[]  SumOutMax=[]  SumI1OutMin=[]  SumI1OutMax=[]  SumI2OutMin=[]  SumI2OutMax=[]  SumI3OutMin=[]  SumI3OutMax=[]  SumDOutMin=[]  SumDOutMax=[]  SaturationOutMin=[]  SaturationOutMax=[]  IntegratorContinuousStateAttributes=''  IntegratorStateMustResolveToSignalObject=off  IntegratorRTWStateStorageClass=Auto  FilterContinuousStateAttributes=''  FilterStateMustResolveToSignalObject=off  FilterRTWStateStorageClass=Auto
  PID braking : simulink_need_slupdate/PID Controller  P=0.3  I=0.01  D=0
  Product : Product
  Product1 : Product
  Product7 : Product
  Relational Operator : RelationalOperator  Operator=>  OutDataTypeStr=boolean
  Saturation : Saturate  UpperLimit=1  LowerLimit=0
  Saturation1 : Saturate  UpperLimit=0  LowerLimit=-1
  Start PID : Subsystem
  Switch : Switch  Threshold=1
  Throttle [Nm] : Outport
  Brake [Nm] : Outport  Port=2
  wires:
  PID braking/1 -> Product1/2
  Product1/1 -> PI1/1(In1), Cockpit1/1
  Add1/1 -> PID braking/1, Switch/3
  v_dem [km/h]/1 -> Add1/1, Relational Operator/2
  v_veh [km/h]/1 -> Add1/2, Relational Operator/1, Compare To Constant3/1
  PID Controller/1 -> Product/2
  Product/1 -> Cockpit/2, Mux/1, Start PID/1(Throttle)
  Logical Operator/1 -> Product/1
  Saturation1/1 -> Cockpit1/3, Brake [Nm]/1, Mux/2
  Product7/1 -> Product1/1, Logical Operator/1
  Compare To Constant3/1 -> Product7/1
  Relational Operator/1 -> Product7/2
  PI1/1(Out1) -> Saturation1/1, Cockpit1/2
  Switch/1 -> PID Controller/1
  Constant/1 -> Switch/1
  Status_Num/1 -> Compare To Constant/1, Compare To Constant1/1
  Compare To Constant/1 -> Logical Operator1/2
  Ground_2/1 -> Cockpit1/4
  Start PID/1(Te_dem) -> Cockpit/3, Saturation/1
  n_eng[rpm]/1 -> Start PID/2(n_eng[rpm]), Cockpit/1
  Saturation/1 -> Cockpit/4, PI/1(In1)
  Compare To Constant1/1 -> Logical Operator1/1, Start PID/3(StatusNum[-])
  Mux/1 -> Cockpit2/1
  Logical Operator1/1 -> Switch/2
  PI/1(Out1) -> Throttle [Nm]/1

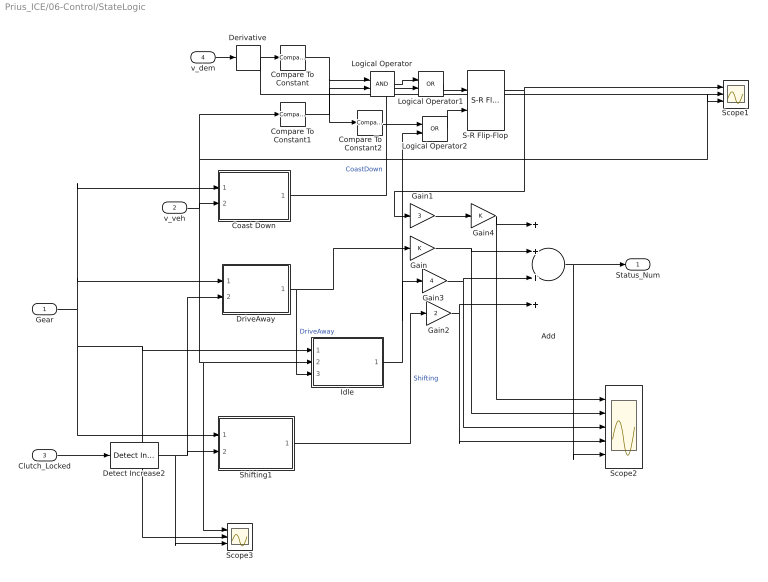
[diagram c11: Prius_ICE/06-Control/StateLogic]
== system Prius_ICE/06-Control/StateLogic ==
  Gear : Inport
  v_veh : Inport  Port=2
  Clutch_Locked : Inport  Port=3
  v_dem : Inport  Port=4
  Add : Sum  Inputs=++++
  Coast Down : Subsystem
  Compare To Constant : simulink/Logic and Bit Operations/Compare To Constant  relop=<  const=0  OutDataTypeStr=uint8
  Compare To Constant1 : simulink/Logic and Bit Operations/Compare To Constant  relop=<=  const=10  OutDataTypeStr=uint8
  Compare To Constant2 : simulink/Logic and Bit Operations/Compare To Constant  relop=>  const=0  OutDataTypeStr=uint8
  Derivative : Derivative
  Detect Increase2 : simulink/Logic and Bit Operations/Detect Increase  vinit=0.0  InputProcessing=Inherited  OutDataTypeStr=boolean
  DriveAway : Subsystem
  Gain : Gain
  Gain1 : Gain  Gain=3
  Gain2 : Gain  Gain=2
  Gain3 : Gain  Gain=4
  Gain4 : Gain
  Idle : Subsystem
  Logical Operator : Logic  AllPortsSameDT=off  OutDataTypeStr=boolean
  Logical Operator1 : Logic  Operator=OR  AllPortsSameDT=off  OutDataTypeStr=boolean
  Logical Operator2 : Logic  Operator=OR  AllPortsSameDT=off  OutDataTypeStr=boolean
  S-R Flip-Flop : simulink_extras/Flip Flops/S-R Flip-Flop  initial_condition=0
  Scope1 : Scope  NumInputPorts=3
  Scope2 : Scope  NumInputPorts=5
  Scope3 : Scope  NumInputPorts=3
  Shifting1 : Subsystem
  Status_Num : Outport
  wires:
  Gear/1 -> Coast Down/1(Gear), DriveAway/1(Gear), Shifting1/1(Gear), Idle/1(Gear), Scope3/2
  v_veh/1 -> Coast Down/2(v_veh), Compare To Constant1/1, Scope1/2, Idle/2(v_veh), Scope3/1
  Clutch_Locked/1 -> Detect Increase2/1
  Detect Increase2/1 -> DriveAway/2(ClutchLocked), Shifting1/2(ClutchLocked), Scope3/3
  DriveAway/1(Drive away) -> Idle/3(Drive_away), Gain/1  "DriveAway"
  Shifting1/1(Shifting) -> Gain2/1  "Shifting"
  Idle/1(Idle) -> Gain3/1, Logical Operator2/2
  Gain/1 -> Add/2, Scope2/2
  Gain1/1 -> Gain4/1
  Gain2/1 -> Add/4, Scope2/4
  Gain3/1 -> Add/3, Scope2/3
  Add/1 -> Status_Num/1, Scope2/5
  Compare To Constant/1 -> Logical Operator/1, Compare To Constant2/1
  Compare To Constant1/1 -> Logical Operator/2
  S-R Flip-Flop/1 -> Scope1/1, Gain1/1
  v_dem/1 -> Derivative/1
  Derivative/1 -> Compare To Constant/1, Scope1/3
  Logical Operator/1 -> Logical Operator1/1
  Logical Operator1/1 -> S-R Flip-Flop/1
  Coast Down/1(Roll off) -> Logical Operator1/2  "CoastDown"
  Gain4/1 -> Add/1, Scope2/1
  Logical Operator2/1 -> S-R Flip-Flop/2
  Compare To Constant2/1 -> Logical Operator2/1

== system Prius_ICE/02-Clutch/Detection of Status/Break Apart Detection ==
  T_ec : Inport
  T_cg : Inport  Port=2
  Tfmaxs : Inport  Port=3
  Abs : Abs
  Mux : Mux  Inputs=2
  Relational Operator : RelationalOperator
  Required Friction Torque : Fcn  Expr=(Clutch.Inp.Inertia*Clutch.Out.Inertia/(Clutch.Inp.Inertia+Clutch.Out.Inertia))*(u(1)/Clutch.Inp.Inertia+u(2)/Clutch.Out.Inertia)
  Break Apart : Outport
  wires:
  Relational Operator/1 -> Break Apart/1
  Tfmaxs/1 -> Relational Operator/2
  Required Friction Torque/1 -> Abs/1
  Mux/1 -> Required Friction Torque/1
  T_ec/1 -> Mux/1
  T_cg/1 -> Mux/2
  Abs/1 -> Relational Operator/1

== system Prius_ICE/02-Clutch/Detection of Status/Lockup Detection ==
  T_ec : Inport
  T_cg : Inport  Port=2
  Tfmaxs : Inport  Port=3
  Count : Inport  Port=4
  " " : Logic  Inputs=3
  Abs : Abs
  Constant : Constant  Value=0.2
  Mux : Mux  Inputs=2
  Mux1 : Mux  Inputs=2
  Mux2 : Mux  Inputs=2
  Relational Operator : RelationalOperator  Operator=<=
  Relational Operator1 : RelationalOperator  OutDataTypeStr=boolean
  Required Friction Torque : Fcn  Expr=(Clutch.Inp.Inertia*Clutch.Out.Inertia/(Clutch.Inp.Inertia+Clutch.Out.Inertia))*(u(1)/Clutch.Inp.Inertia+u(2)/Clutch.Out.Inertia)
  Scope1 : Scope
  Scope2 : Scope
  Scope3 : Scope
  Speed Match : HitCross
  Sum : Sum  Inputs=|+-
  Lock Up : Outport
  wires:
  Relational Operator1/1 -> " "/3
  Constant/1 -> Relational Operator1/2
  Count/1 -> Scope3/1, Relational Operator1/1
  Mux2/1 -> Scope1/1
  Mux1/1 -> Scope2/1
  Speed Match/1 -> " "/2
  Mux/1 -> Required Friction Torque/1
  T_ec/1 -> Mux/1
  T_cg/1 -> Mux/2
  " "/1 -> Lock Up/1  "lockup"
  Required Friction Torque/1 -> Mux1/1, Abs/1
  [unlocked_we] -> Sum/1, Mux2/1
  Sum/1 -> Speed Match/1
  Abs/1 -> Relational Operator/1
  Tfmaxs/1 -> Mux1/2, Relational Operator/2
  Relational Operator/1 -> " "/1
  [unlocked_wv] -> Mux2/2, Sum/2

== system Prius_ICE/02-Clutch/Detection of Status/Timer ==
  Set : Inport
  Add1 : Sum  Inputs=-+
  Clock : Clock
  Memory : Memory
  Switch1 : Switch  Threshold=1
  Count : Outport
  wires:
  Set/1 -> Switch1/2
  Add1/1 -> Count/1
  Clock/1 -> Switch1/3, Add1/2
  Memory/1 -> Switch1/1, Add1/1
  Switch1/1 -> Memory/1

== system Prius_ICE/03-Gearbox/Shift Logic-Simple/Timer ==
  Set : Inport
  Reset : Inport  Port=2
  Add1 : Sum  Inputs=-+
  Clock : Clock
  Memory : Memory
  S-R Flip-Flop : simulink_extras/Flip Flops/S-R Flip-Flop  initial_condition=0
  Switch1 : Switch  Threshold=1
  Terminator_1 : Terminator
  Count : Outport
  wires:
  S-R Flip-Flop/2 -> Terminator_1/1
  Reset/1 -> S-R Flip-Flop/2
  S-R Flip-Flop/1 -> Switch1/2
  Set/1 -> S-R Flip-Flop/1
  Add1/1 -> Count/1
  Clock/1 -> Switch1/3, Add1/2
  Memory/1 -> Switch1/1, Add1/1
  Switch1/1 -> Memory/1

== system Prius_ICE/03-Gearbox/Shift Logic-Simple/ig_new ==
  ig : Inport
  Trigger : TriggerPort
  Data Store Write1 : DataStoreWrite  DataStoreName=ig_new
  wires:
  ig/1 -> Data Store Write1/1

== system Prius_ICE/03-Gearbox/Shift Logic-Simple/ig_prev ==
  ig : Inport
  Trigger : TriggerPort
  Data Store Write1 : DataStoreWrite  DataStoreName=ig_prev
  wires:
  ig/1 -> Data Store Write1/1

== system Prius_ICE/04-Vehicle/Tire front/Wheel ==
  F_tire : Inport
  T_drsft : Inport  Port=2
  "        " : Gain  Gain=2*Vehicle.Tyre.Front.Rdyn
  " Inertia Wheel" : Gain  Gain=1/(2*Vehicle.Tyre.Rear.Inertia)
  Sum10 : Sum  Inputs=|-|+|
  "to Rot Speed     " : Integrator  InitialCondition=omric
  om_wheel : Outport
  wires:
  Sum10/1 -> " Inertia Wheel"/1
  " Inertia Wheel"/1 -> "to Rot Speed     "/1
  F_tire/1 -> "        "/1
  T_drsft/1 -> Sum10/2  "T_drv_sft"
  "        "/1 -> Sum10/1  "T_tire"
  "to Rot Speed     "/1 -> om_wheel/1  "om_wheel [rad/s]"

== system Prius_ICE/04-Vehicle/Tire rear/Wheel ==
  F_tire : Inport
  T_drsft : Inport  Port=2
  "        " : Gain  Gain=2*Vehicle.Tyre.Front.Rdyn
  " Inertia Wheel" : Gain  Gain=1/(2*Vehicle.Tyre.Front.Inertia)
  Sum10 : Sum  Inputs=|-|+|
  "to Rot Speed     " : Integrator  InitialCondition=omric
  om_wheel : Outport
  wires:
  "to Rot Speed     "/1 -> om_wheel/1  "om_wheel [rad/s]"
  "        "/1 -> Sum10/1  "T_tire"
  T_drsft/1 -> Sum10/2  "T_drv_sft"
  F_tire/1 -> "        "/1
  " Inertia Wheel"/1 -> "to Rot Speed     "/1
  Sum10/1 -> " Inertia Wheel"/1

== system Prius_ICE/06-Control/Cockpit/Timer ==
  Set : Inport
  Add1 : Sum  Inputs=-+
  Clock : Clock
  Memory : Memory
  Switch1 : Switch  Threshold=1
  Count : Outport
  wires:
  Switch1/1 -> Memory/1
  Memory/1 -> Add1/1, Switch1/1
  Clock/1 -> Add1/2, Switch1/3
  Add1/1 -> Count/1
  Set/1 -> Switch1/2

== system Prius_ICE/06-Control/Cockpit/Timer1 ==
  Set : Inport
  Add1 : Sum  Inputs=-+
  Clock : Clock
  Memory : Memory
  Switch1 : Switch  Threshold=1
  Count : Outport
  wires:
  Set/1 -> Switch1/2
  Add1/1 -> Count/1
  Clock/1 -> Switch1/3, Add1/2
  Memory/1 -> Switch1/1, Add1/1
  Switch1/1 -> Memory/1
